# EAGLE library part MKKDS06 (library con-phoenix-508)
PHOENIX
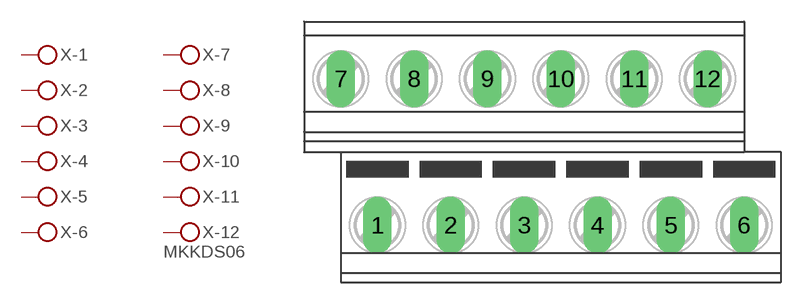
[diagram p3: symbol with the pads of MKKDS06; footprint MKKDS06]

Designator prefix X; gates -1=KL -2=KL -3=KL -4=KL -5=KL -6=KL -7=KL -8=KL -9=KL -10=KL -11=KL -12=KLV

## MKKDS06 (OC_FARNELL: unknown; OC_NEWARK: unknown)  [MKKDS06]
1  -1:KL  pas
2  -2:KL  pas
3  -3:KL  pas
4  -4:KL  pas
5  -5:KL  pas
6  -6:KL  pas
7  -7:KL  pas
8  -8:KL  pas
9  -9:KL  pas
10  -10:KL  pas
11  -11:KL  pas
12  -12:KL  pas

## Footprint MKKDS06 (pad centres in mm)
PHOENIX MKKDSN 1,5/ 8-5,08 Source: http://eshop.phoenixcontact.com .. 1726202.pdf
drill 1.321 long: 1 -11.43,-5.08; 2 -6.35,-5.08; 3 -1.27,-5.08; 4 3.81,-5.08; 5 8.89,-5.08; 6 13.97,-5.08; 7 -13.97,5.08; 8 -8.89,5.08; 9 -3.81,5.08; 10 1.27,5.08; 11 6.35,5.08; 12 11.43,5.08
